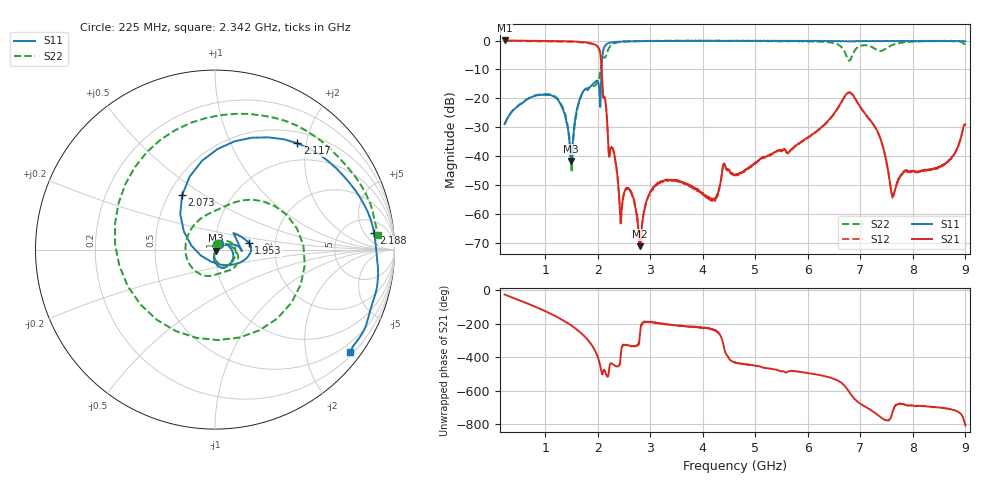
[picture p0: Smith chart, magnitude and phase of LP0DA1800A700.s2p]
!Agilent Technologies,E8358A,US41080443,A.07.50.56
!Agilent E8358A: A.07.50.56
!Date: Wednesday, August 24, 2016 14:36:46
!Correction: S11(Full 2 Port(1,2))
!S21(Full 2 Port(1,2))
!S12(Full 2 Port(1,2))
!S22(Full 2 Port(1,2))
!S2P File: Measurements: S11, S21, S12, S22:
# Hz S  dB  R 50
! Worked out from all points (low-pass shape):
!   1601 points, 225 MHz to 9 GHz, reference 50 ohm
!   highest |S21| = 0.04 dB at 225 MHz (marker M1); lowest = -71.2 dB at 2.803 GHz (marker M2)
!   |S21| within 3 dB of the highest: start of sweep to 2.027 GHz
!   lowest |S11| = -41.7 dB at 1.492 GHz (marker M3), VSWR 1.02, Z = 50.6 - j0.52 ohm
!   |S11| at or under -10 dB: start of sweep to 2.071 GHz
!   |S22| runs from -45.6 to 0.0 dB; largest |S21 - S12| = 0.019
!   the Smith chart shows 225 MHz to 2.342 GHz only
!   S11 on the Smith chart (normalised r, x): 225 MHz: 1.04, +0.06; 1.953 GHz: 1.46, +0.12; 2.073 GHz: 0.59, +0.41; 2.117 GHz: 0.68, +1.84; 2.188 GHz: 10, +9; 2.342 GHz: 0.28, -2.96
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2.25e8  -28.95 55.9  0.04 -27.0  -0.12 -26.7  -28.91 70.3
8.721562e8  -18.90 -32.3  -0.12 -108.4  -0.27 -108.1  -18.71 -4.4
1.491891e9  -41.68 -38.5  -0.26 149.0  -0.41 149.2  -42.62 -74.7
1.689328e9  -18.75 13.2  -0.50 100.8  -0.64 101.0  -18.93 -1.2
1.952578e9  -14.32 11.5  -1.44 -5.3  -1.58 -5.1  -15.50 161.3
2.073234e9  -9.00 121.1  -9.66 -134.9  -9.84 -134.6  -7.04 25.7
2.117109e9  -2.50 52.2  -19.43 -115.0  -19.62 -114.9  -5.87 -74.4
2.188406e9  -1.00 5.9  -31.70 -157.2  -31.85 -156.7  -3.57 125.0
2.341969e9  -0.50 -37.1  -42.24 -93.6  -42.55 -94.4  -0.82 5.3
2.802656e9  -0.18 -89.2  -71.20 99.5  -70.24 103.4  -0.17 -78.0
3.153656e9  -0.15 -109.0  -49.53 163.4  -49.28 161.0  -0.10 -105.1
4.6125e9  -0.13 -142.3  -46.53 -71.2  -46.61 -73.1  -0.12 -179.4
6.076828e9  -0.06 -168.1  -32.50 -139.7  -32.77 -139.7  -0.35 79.3
6.603328e9  -0.13 179.4  -22.31 173.4  -22.56 174.2  -1.76 7.4
6.740438e9  -0.22 176.1  -18.37 132.5  -18.50 133.2  -5.64 -72.1
6.850125e9  -0.18 174.9  -18.65 84.3  -18.82 84.4  -4.93 154.5
6.998203e9  -0.15 170.7  -22.93 41.2  -23.13 41.6  -1.90 76.7
7.217578e9  -0.20 165.9  -28.29 0.5  -28.31 0.4  -2.15 3.3
7.382109e9  -0.09 162.6  -33.84 -38.1  -34.04 -37.7  -3.62 -89.3
7.541156e9  -0.24 158.7  -46.62 -56.0  -46.64 -56.8  -2.19 -177.0
7.985391e9  -0.16 150.2  -45.11 31.0  -45.40 31.1  -0.42 104.6
9e9  -0.23 131.8  -29.10 -88.1  -29.25 -88.6  -1.28 59.0
